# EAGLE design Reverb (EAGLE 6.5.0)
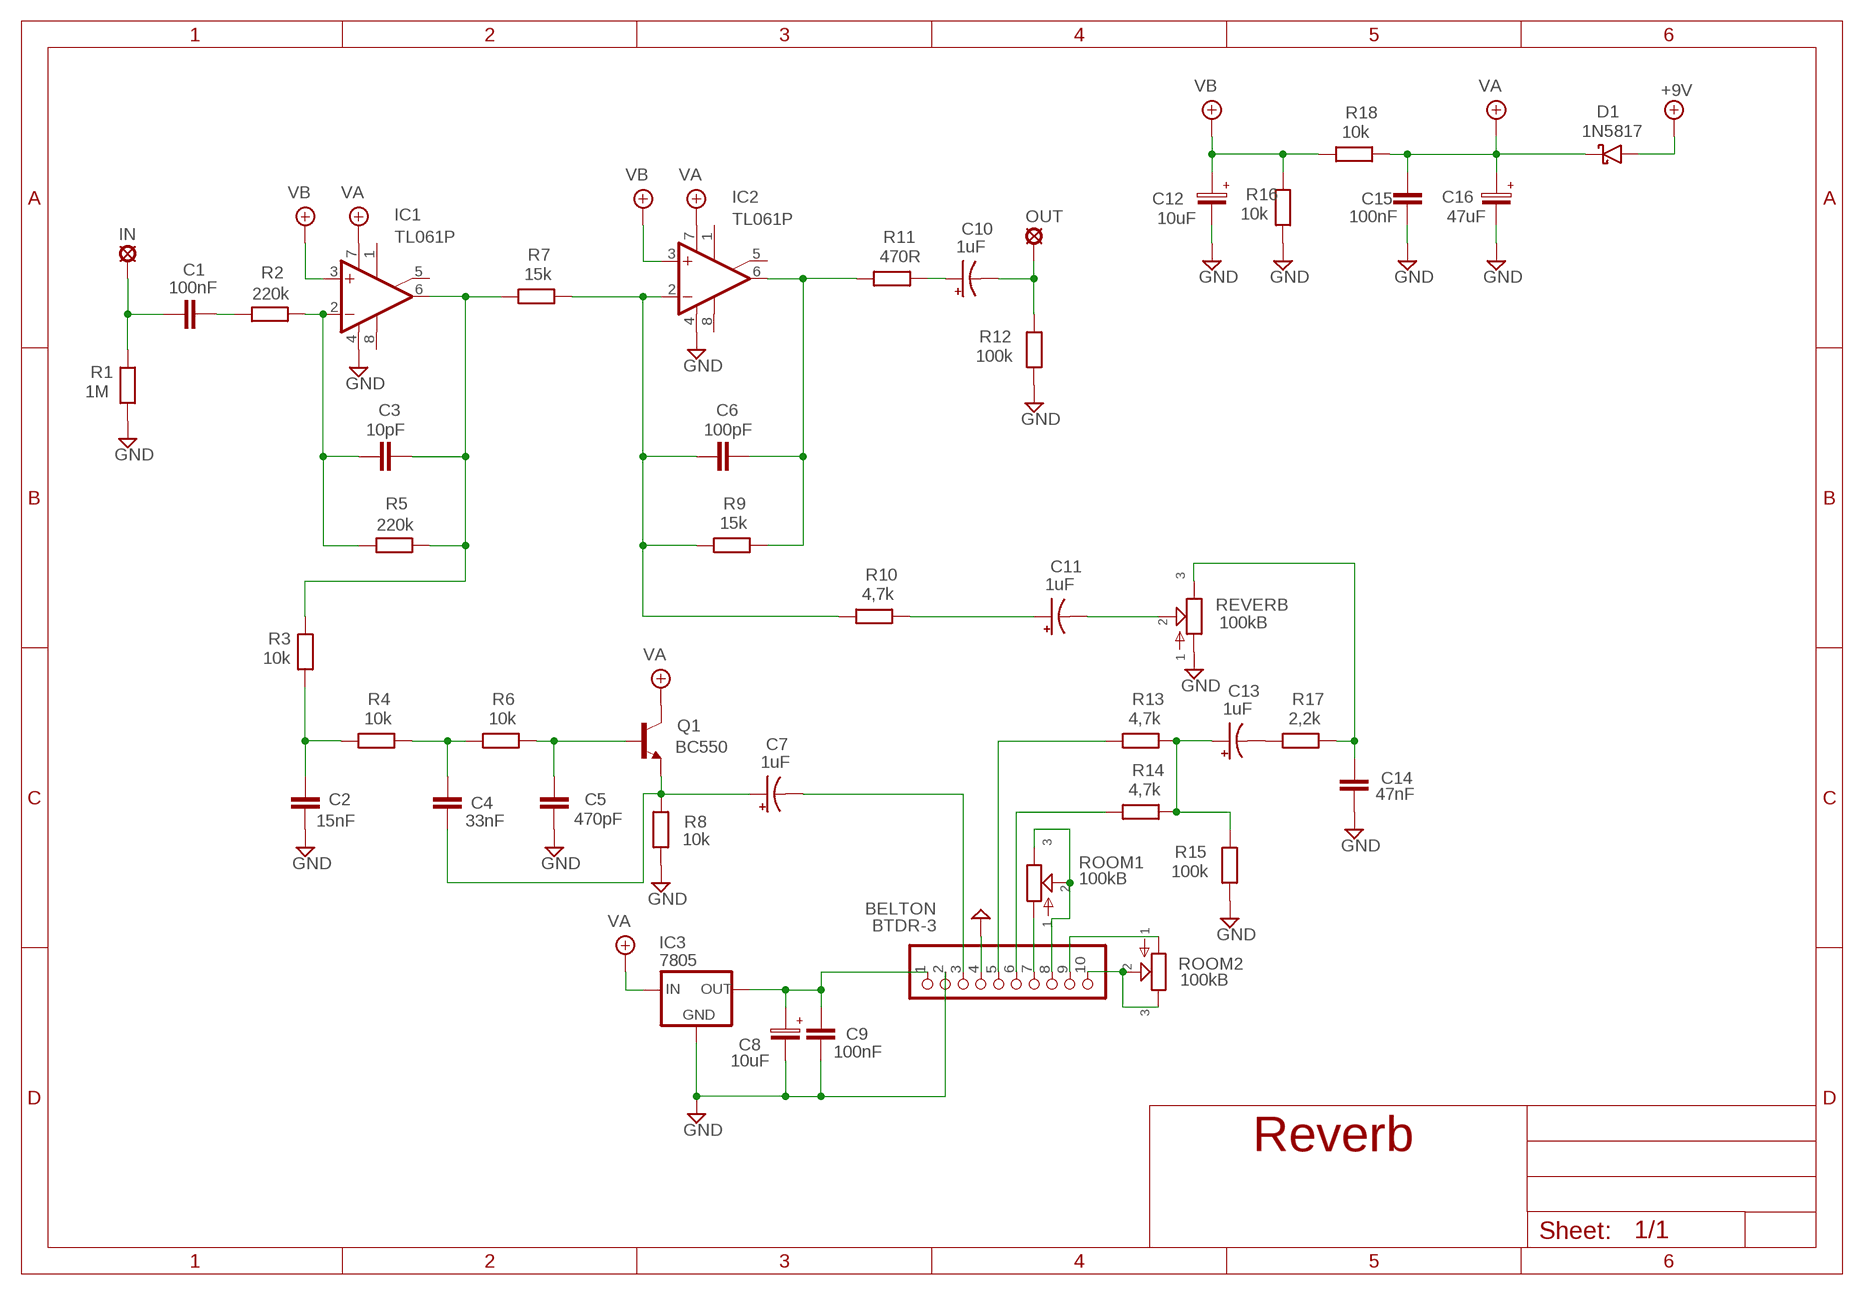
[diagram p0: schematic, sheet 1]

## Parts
+9V  +9V  +9V(T)1  [ROUND]
BTDR-3  BELTON  PINHD-1X10  [1X10]
C1  100nF  100NF-220NF  [7,5MM]
C2  15nF  1NF-15NF  [3,5MM]
C3  10pF  050X030_0251  [050X030_025]
C4  33nF  22NF-82NF"  [4,5MM]
C5  470pF  050X030_0251  [050X030_025]
C6  100pF  050X030_0251  [050X030_025]
C7  1uF  044A1  [044A]
C8  10uF  063-EU  [063_025]
C9  100nF  100NF-220NF  [7,5MM]
C10  1uF  044A1  [044A]
C11  1uF  044A1  [044A]
C12  10uF  063-EU  [063_025]
C13  1uF  044A1  [044A]
C14  47nF  22NF-82NF"  [4,5MM]
C15  100nF  100NF-220NF  [7,5MM]
C16  47uF  063-EU  [063_025]
D1  1N5817  [DO41-3]
GND  GND  GND(T)1  [ROUND]
GND16  GND  GND(T)1  [ROUND]
IC1  TL061P  TL071D  [SO08]
IC2  TL061P  TL071D  [SO08]
IC3  7805  78LXX  [78LXX]
IN  MCS10B  [MCS10B]
OUT  MCS10B  [MCS10B]
Q1  BC550  [TO92-]
R1  1M  6MM-EU3  [R0207/3]
R2  220k  6MM-EU3  [R0207/3]
R3  10k  6MM-EU3  [R0207/3]
R4  10k  6MM-EU3  [R0207/3]
R5  220k  6MM-EU3  [R0207/3]
R6  10k  6MM-EU3  [R0207/3]
R7  15k  6MM-EU3  [R0207/3]
R8  10k  6MM-EU3  [R0207/3]
R9  15k  6MM-EU3  [R0207/3]
R10  4,7k  6MM-EU3  [R0207/3]
R11  470R  6MM-EU3  [R0207/3]
R12  100k  6MM-EU3  [R0207/3]
R13  4,7k  6MM-EU3  [R0207/3]
R14  4,7k  6MM-EU3  [R0207/3]
R15  100k  6MM-EU3  [R0207/3]
R16  10k  6MM-EU3  [R0207/3]
R17  2,2k  6MM-EU3  [R0207/3]
R18  10k  6MM-EU3  [R0207/3]
REVERB  100kB  POT-EU16MM  [16MM]
ROOM1  100kB  POT-EU16MM  [16MM]
ROOM2  100kB  POT-EU16MM  [16MM]

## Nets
+9V: +9V.1(+9V) D1.A
GND: BTDR-3.2 BTDR-3.4 C2.2 C5.2 C8.- C9.P$2 C12.- C14.2 C15.P$2 C16.- GND16.1(GND) GND.1(GND) IC1.4(V-) IC2.4(V-) IC3.GND R1.2 R8.2 R12.2 R15.2 R16.2 REVERB.1
N$1: C3.1 IC1.2(-IN) R2.2 R5.1
N$2: C1.P$2 R2.1
N$3: C1.P$1 IN.MP R1.1
N$4: C3.2 IC1.6(OUT) R3.1 R5.2 R7.1
N$5: C6.1 IC2.2(-IN) R7.2 R9.1 R10.1
N$6: C10.1(+) R11.2
N$7: C6.2 IC2.6(OUT) R9.2 R11.1
N$8: C10.2(-) OUT.MP R12.1
N$9: BTDR-3.9 ROOM2.1
N$10: BTDR-3.6 R14.1
N$11: BTDR-3.7 ROOM1.1
N$12: BTDR-3.8 ROOM1.2 ROOM1.3
N$13: BTDR-3.1 C8.+ C9.P$1 IC3.OUT
N$14: C4.2 C7.1(+) Q1.1(E) R8.1
N$15: BTDR-3.3 C7.2(-)
N$16: BTDR-3.10 ROOM2.2 ROOM2.3
N$17: C4.1 R4.2 R6.1
N$18: C5.1 Q1.2(B) R6.2
N$19: C2.1 R3.2 R4.1
N$20: BTDR-3.5 R13.1
N$21: C13.1(+) R13.2 R14.2 R15.1
N$22: C13.2(-) R17.1
N$23: C14.1 R17.2 REVERB.3
N$24: C11.2(-) REVERB.2
N$25: C11.1(+) R10.2
VA: C15.P$1 C16.+ D1.C IC1.7(V+) IC2.7(V+) IC3.IN Q1.3(C) R18.2
VB: C12.+ IC1.3(+IN) IC2.3(+IN) R16.1 R18.1
Unconnected: IC1.1(ON1) IC1.5(ON2) IC1.8(OPT) IC2.1(ON1) IC2.5(ON2) IC2.8(OPT)

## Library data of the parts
+9V = gm-supply:+9V(T): +9V Voltage Supply
BTDR-3 = pinhead:PINHD-1X10: PIN HEADER
C1 C9 C15 = Mylar Kondensaattorit:100NF-220NF: 100nF-220nF
C2 = Mylar Kondensaattorit:1NF-15NF: 1nF-15nF
C3 C5 C6 = Keraamiset kondensaattorit:050X030_025: 47 - 120pF
C4 C14 = Mylar Kondensaattorit:22NF-82NF: 22nF-82nF
C7 C10 C11 C13 = Tantaalit:044A: .1 - 1.5µF
C8 C12 C16 = Elektrolyytit:063-EU
D1 = Diodit:1N5817
GND GND16 = gm-supply:GND(T): Ground
IC1 IC2 = Operaatiovahvistimet:TL071: OP AMP
IC3 = v-reg:78LXX: VOLTAGE REGULATOR
IN OUT = Padit:MCS10B: SOLDER PAD
Q1 = Transistorit:BC550
R1-R18 = Vastukset:6MM-EU: 6mm Resistors (European schematic symbol)
REVERB ROOM1 ROOM2 = gm-pots:POT-EU

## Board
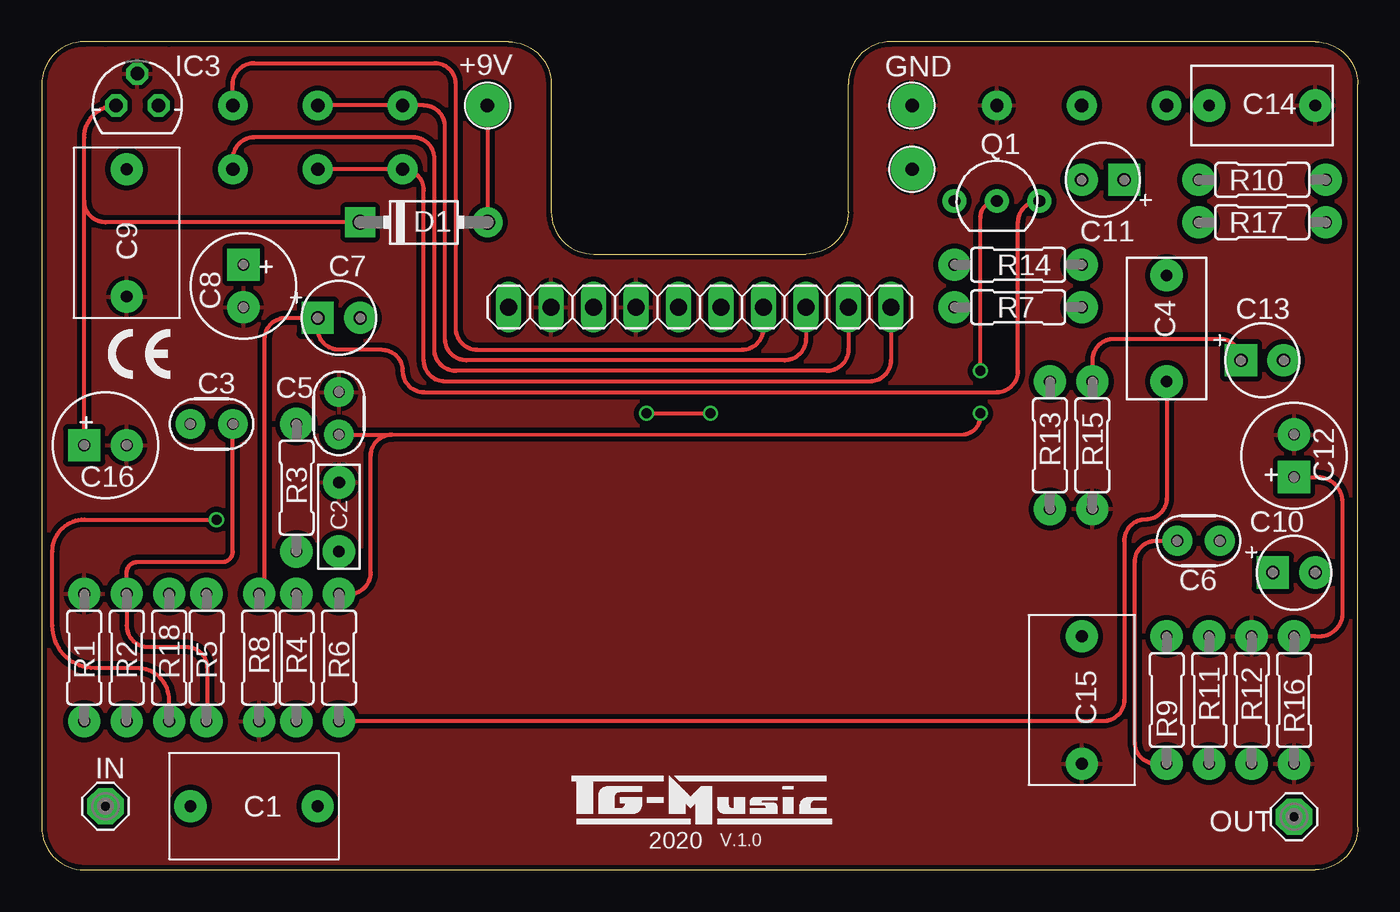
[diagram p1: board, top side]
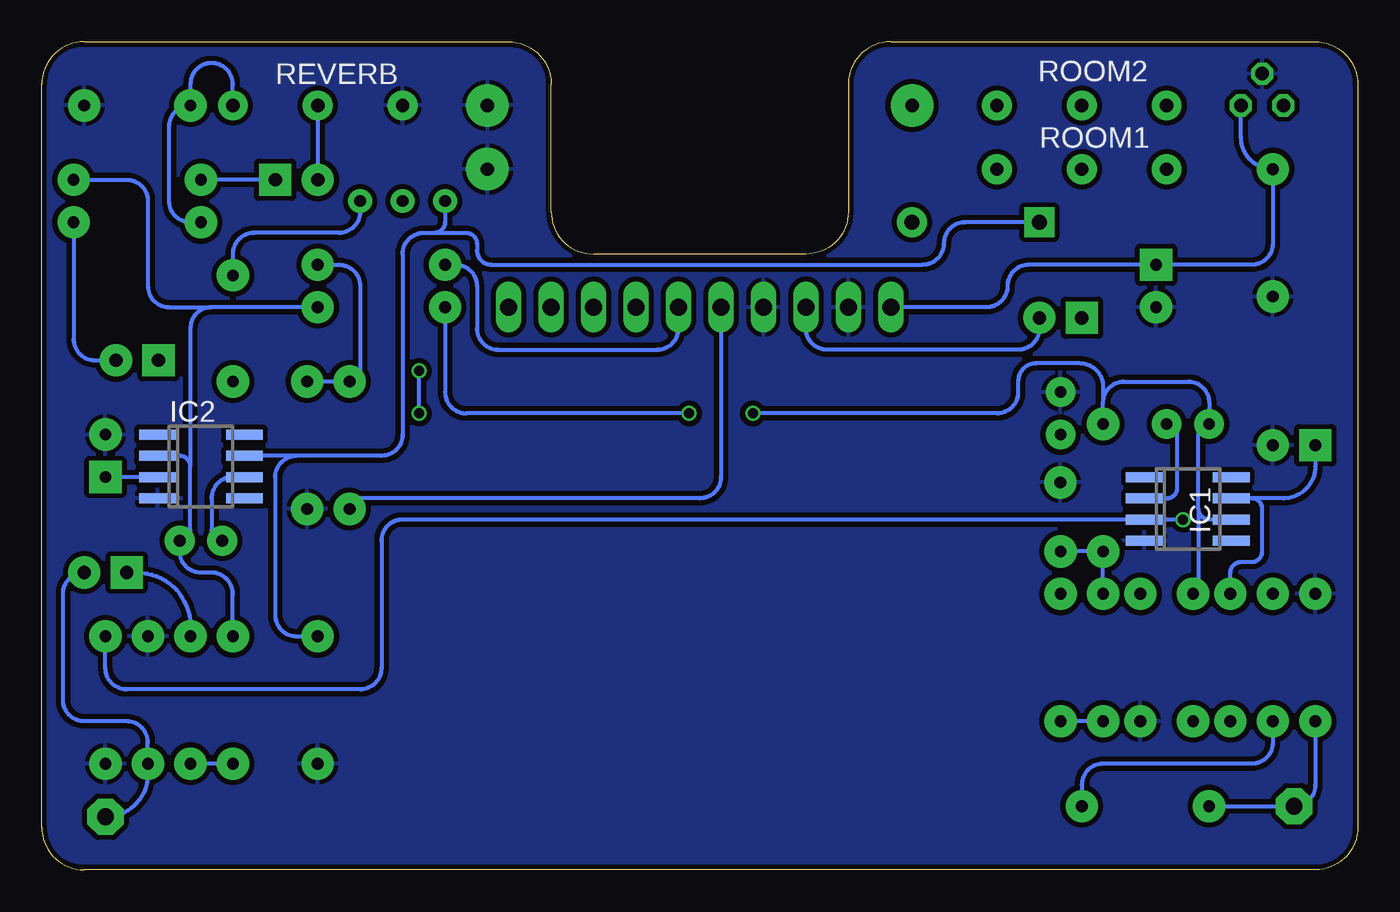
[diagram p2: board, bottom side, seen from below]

Size 78.74 x 49.53 mm. Coordinates in mm from the lower left corner, seen from the top.
Outline: 7.62,49.53 3.81,49.53
Outline: 78.74,2.54 78.74,46.99 arc90 76.2,49.53 50.8,49.53 arc90 48.26,46.99 48.26,39.37 arc-90 45.72,36.83 33.02,36.83 arc-90 30.48,39.37 30.48,46.99 arc90 27.94,49.53 2.54,49.53 arc90 0,46.99 0,2.54 arc90 2.54,0 76.2,0 arc90 78.74,2.54
Copper layers (1*16): Top 0.035mm / dielectric 1.5mm / Bottom 0.035mm
Design rules "ITEADstudio": minimum track width 10mil, minimum drill 12mil, track to track 12mil, track to pad 12mil, pad to pad 12mil, via to via 12mil, smd to smd 0mil, copper to edge 12mil, drill to drill 12mil, minimum pad ring 10mil, minimum via ring 6mil, stop-mask expansion 4mil, vias tented up to drill 100mil, thermal gap 10mil

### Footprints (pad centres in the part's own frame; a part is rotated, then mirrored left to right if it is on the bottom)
ROUND = drill 0.8 pad 2.54: 1 0,0
1X10 = drill 1.016 long: 1 -11.43,0; 2 -8.89,0; 3 -6.35,0; 4 -3.81,0; 5 -1.27,0; 6 1.27,0; 7 3.81,0; 8 6.35,0; 9 8.89,0; 10 11.43,0
7,5MM = drill 0.7 pad 1.93: P$1 -3.81,0; P$2 3.81,0
3,5MM = drill 0.7 pad 1.93: 1 -1.905,0; 2 2.221,-0.016
050X030_025 = drill 0.7 pad 1.778: 1 -1.27,0; 2 1.27,0
4,5MM = drill 0.7 pad 1.93: 1 -3.175,0; 2 3.175,0
044A = drill 0.8 pad 1.93 square: 1 -1.27,0 | drill 0.8 pad 1.93: 2 1.27,0
063_025 = drill 0.7 pad 1.93 square: + -1.27,0 | drill 0.7 pad 1.93: - 1.27,0
DO41-3 = drill 0.9 pad 1.778: A 3.81,0 | drill 0.9 pad 1.778 square: C -3.81,0
SO08 = smd 0.6 x 2.2: 1 -1.905,-2.6; 2 -0.635,-2.6; 3 0.635,-2.6; 4 1.905,-2.6; 5 1.905,2.6; 6 0.635,2.6; 7 -0.635,2.6; 8 -1.905,2.6
78LXX = drill 0.813 octagon: GND 0,1.905; IN -1.27,0; OUT 1.27,0
MCS10B = drill 1.016 pad 2.159 octagon: MP 0,0
TO92- = drill 0.7 pad 1.422: 1 2.54,0; 2 0,0; 3 -2.54,0
R0207/3 = drill 0.7 pad 1.93: 1 -3.81,0; 2 3.81,0
16MM = drill 0.8 pad 1.778: 1 5.08,0; 2 0,0; 3 -5.08,0

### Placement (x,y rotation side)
+9V  26.67,45.72 0 top
BTDR-3  39.37,33.66 0 top
C1  12.7,3.81 0 top
C2  17.78,20.95 90 top
C3  10.16,26.67 180 top
C4  67.31,32.38 90 top
C5  17.78,27.3 90 top
C6  69.22,19.68 180 top
C7  17.78,33.02 0 top
C8  12.06,34.92 270 top
C9  5.08,38.1 270 top
C10  74.93,17.78 0 top
C11  63.5,41.27 180 top
C12  74.93,24.77 90 top
C13  73.03,30.48 0 top
C14  73.03,45.72 0 top
C15  62.23,10.16 270 top
C16  3.81,25.4 0 top
D1  22.86,38.73 0 top
GND  52.07,45.72 0 top
GND16  52.07,41.91 0 top
IC1  10.16,21.59 270 bottom
IC2  69.22,24.13 270 bottom
IC3  5.71,45.72 0 top
IN  3.81,3.81 0 top
OUT  74.93,3.17 0 top
Q1  57.15,40.01 0 top
R1  2.54,12.7 90 top
R2  5.08,12.7 90 top
R3  15.24,22.86 270 top
R4  15.24,12.7 270 top
R5  9.86,12.7 90 top
R6  17.78,12.7 90 top
R7  58.42,33.66 0 top
R8  13,12.7 270 top
R9  67.31,10.16 270 top
R10  73.03,41.27 180 top
R11  69.85,10.16 90 top
R12  72.39,10.16 90 top
R13  60.33,25.4 90 top
R14  58.42,36.2 0 top
R15  62.87,25.4 270 top
R16  74.93,10.16 270 top
R17  73.03,38.73 180 top
R18  7.62,12.7 90 top
REVERB  62.23,45.72 0 bottom
ROOM1  16.51,45.72 0 bottom
ROOM2  16.51,41.91 0 bottom

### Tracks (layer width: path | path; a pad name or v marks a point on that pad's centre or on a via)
+9V
  Top 0.254: +9V.1 D1.A
GND
  pour Bottom: 0,1.91 0,46.99 arc-90 2.54,49.53 27.94,49.53 arc-90 30.48,46.99 30.48,39.37 arc90 33.02,36.83 45.09,36.83 arc90 48.26,40.01 48.26,46.99 arc-90 50.8,49.53 75.56,49.53 arc-90 78.74,46.35 78.74,2.54 arc-90 76.2,0 1.91,0 arc-90
  pour Top: 0,1.27 0,46.99 arc-90 2.54,49.53 27.94,49.53 arc-90 30.48,46.99 30.48,39.37 arc90 33.02,36.83 45.09,36.83 arc90 48.26,40.01 48.26,46.35 arc-90 51.44,49.53 75.56,49.53 arc-90 78.74,46.35 78.74,1.91 arc-90 76.83,0 1.27,0 arc-90
N$1
  Top 0.254: C3.1 11.43,19.05 arc-90 10.79,18.41 5.71,18.41 arc90 5.08,17.78 R2.2 5.08,14.61 arc90 6.35,13.34 8.66,13.34 arc-90 9.89,12.11 9.89,8.92 arc-90 R5.1
  Bottom 0.254: IC1.2 11.43,22.23 arc-90 10.79,22.86 10.79,26.04 arc-90 C3.1
N$2
  Bottom 0.254: R2.1 5.08,7.62 arc90 6.35,6.35 15.24,6.35 arc-90 16.51,5.08 C1.P$2
N$3
  Bottom 0.254: C1.P$1 IN.MP arc-90 2.54,5.08 R1.1
N$4  (via drill 0.6)
  Top 0.254: v36.2,27.3 v40.01,27.3
  Bottom 0.254: IC1.6 8.89,20.95 arc90 9.53,21.59 | 9.53,21.59 9.53,26.04 arc90 C3.2 8.89,27.94 arc-90 10.16,29.21 13.97,29.21 arc-90 15.24,27.94 | R5.2 arc-90 9.53,17.14 9.53,21.59 | R7.1 54.61,28.57 arc-90 53.34,27.3 v40.01,27.3 | R3.1 15.24,27.94 | v36.2,27.3 21.59,27.3 arc-90 20.32,28.57 20.32,29.21 arc90 19.23,30.3 16.62,30.3 arc90 15.24,28.91 15.24,27.94 arc90 15.24,27.94
N$5
  Bottom 0.254: 69.85,24.13 69.85,20.32 arc90 C6.1 70.48,19.05 arc-90 69.22,17.78 68.58,17.78 arc90 67.31,16.51 R9.1 | 69.85,24.13 arc-90 70.48,24.77 IC2.2 | R7.2 68.58,33.66 | 68.58,33.66 arc-90 69.85,32.38 69.85,24.13 | R10.1 73.66,41.27 arc90 72.39,40.01 72.39,34.92 arc-90 71.12,33.66 68.58,33.66
N$6
  Bottom 0.254: C10.1 73.03,17.78 arc90 69.85,14.61 R11.2
N$7
  Top 0.254: R9.2 66.67,6.35 arc-90 65.41,7.62 65.41,18.41 arc-90 66.67,19.68 C6.2
  Bottom 0.254: IC2.6 67.31,23.5 arc-90 68.58,22.23 68.58,20.32 arc-90 C6.2 | R9.2 R11.1
N$8
  Bottom 0.254: OUT.MP arc-90 72.39,5.71 R12.1 72.39,7.62 arc-90 73.66,8.89 76.2,8.89 arc90 77.47,10.16 77.47,16.51 arc90 C10.2
N$9
  Top 0.254: BTDR-3.9 48.26,31.11 arc-90 46.99,29.84 24.77,29.84 arc-90 23.5,31.11 23.5,42.55 arc90 22.23,43.81 12.7,43.81 arc90 11.43,42.55 ROOM2.1
N$10
  Bottom 0.254: BTDR-3.6 40.64,32.38 arc90 41.91,31.11 51.44,31.11 arc90 52.7,32.38 52.7,34.92 arc-90 53.98,36.2 R14.1
N$11
  Top 0.254: ROOM1.1 11.43,46.99 arc-90 12.7,48.26 23.5,48.26 arc-90 24.77,46.99 24.77,32.38 arc90 26.04,31.11 41.91,31.11 arc90 43.18,32.38 BTDR-3.7
N$12
  Top 0.254: BTDR-3.8 45.72,31.75 arc-90 44.45,30.48 25.4,30.48 arc-90 24.13,31.75 24.13,44.45 arc90 22.86,45.72 ROOM1.3 ROOM1.2
N$13
  Bottom 0.254: BTDR-3.1 22.23,33.66 arc-90 20.95,34.92 arc90 19.68,36.2 C8.+ 6.35,36.2 arc-90 5.08,37.47 C9.P$1 arc90 6.99,43.81 IC3.OUT
N$14
  Top 0.254: R8.1 arc90 13.34,17.14 13.34,31.75 arc-90 14.61,33.02 C7.1 16.51,32.38 arc90 17.78,31.11 20.32,31.11 arc-90 21.59,29.84 arc90 22.86,28.57 57.15,28.57 arc90 58.42,29.84 58.42,38.73 arc-90 Q1.1
  Bottom 0.254: Q1.1 59.69,39.37 arc90 60.96,38.1 66.04,38.1 arc-90 67.31,36.83 C4.2
N$15
  Bottom 0.254: C7.2 19.05,32.38 arc90 20.32,31.11 31.75,31.11 arc90 33.02,32.38 BTDR-3.3
N$16
  Top 0.254: BTDR-3.10 50.8,30.48 arc-90 49.53,29.21 24.13,29.21 arc-90 22.86,30.48 22.86,40.64 arc90 ROOM2.3 ROOM2.2
N$17
  Top 0.254: C4.1 67.31,22.23 arc-90 66.04,20.95 arc90 64.77,19.68 64.77,10.16 arc-90 63.5,8.89 R6.1
  Bottom 0.254: R4.2 R6.1
N$18  (via drill 0.6)
  Top 0.254: C5.1 20.95,26.04 | 20.95,26.04 55.2,26.05 arc90 v56.16,27.3 | v56.16,29.84 56.16,39.02 arc-90 Q1.2 | R6.2 18.41,16.51 arc90 19.68,17.78 19.68,24.77 arc-90 20.95,26.04
  Bottom 0.254: v56.16,27.3 v56.16,29.84
N$19
  Bottom 0.254: R4.1 R3.2 C2.1
N$20
  Bottom 0.254: BTDR-3.5 38.1,23.5 arc90 39.37,22.23 59.69,22.23 arc-90 R13.1
N$21
  Top 0.254: C13.1 arc90 70.48,31.75 64.14,31.75 arc90 62.87,30.48 R15.1
  Bottom 0.254: R15.1 R13.2 arc-90 59.69,29.84 59.69,34.92 arc-90 60.96,36.2 R14.2
N$22
  Bottom 0.254: R17.1 76.83,31.75 arc-90 75.56,30.48 C13.2
N$23
  Bottom 0.254: R17.2 69.85,38.73 arc90 71.12,40.01 71.12,44.45 arc90 C14.1 69.85,46.99 arc90 68.58,48.26 arc90 67.31,46.99 REVERB.3
N$24
  Bottom 0.254: REVERB.2 C11.2
N$25
  Bottom 0.254: C11.1 R10.2
VA
  Top 0.254: D1.C 3.81,38.73 arc-90 2.54,40.01 | C16.+ 2.54,40.01 | 2.54,40.01 2.54,43.81 arc-90 IC3.IN
  Bottom 0.254: C16.+ 2.54,24.13 arc90 4.45,22.23 6.35,22.23 | 6.35,22.23 IC1.7 | R18.2 7.62,17.78 arc90 6.99,18.41 6.35,18.41 arc-90 5.71,19.05 5.71,21.59 arc-90 6.35,22.23 | C15.P$1 63.5,13.97 arc90 64.77,15.24 64.77,23.5 arc90 63.5,24.77 | 63.5,24.77 58.42,24.77 arc-90 57.15,26.04 57.15,36.83 arc90 55.88,38.1 55.24,38.1 | 63.5,24.77 IC2.7 | D1.C 23.5,38.73 arc-90 24.77,37.47 arc90 26.04,36.2 51.84,36.2 arc90 52.7,37.06 52.7,37.47 arc-90 53.34,38.1 55.24,38.1 | Q1.3 54.61,38.73 arc90 55.24,38.1
VB  (via drill 0.6)
  Top 0.254: C12.+ 76.2,23.5 arc-90 77.81,22.13 77.81,15.14 arc-90 76.2,13.97 R16.1 | R18.1 7.62,10.16 arc90 5.71,12.06 3.17,12.06 arc-90 0.64,14.61 0.64,19.05 arc-90 2.54,20.95 v10.45,20.95 arc-90 v10.45,20.95
  Bottom 0.254: v10.45,20.95 IC1.3 arc90 IC1.3 57.15,20.95 arc-90 58.42,19.68 58.42,12.06 arc90 59.69,10.79 73.66,10.79 arc90 74.93,12.06 R16.1 | IC2.3 C12.+

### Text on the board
tNames: 2020 | V.1.0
